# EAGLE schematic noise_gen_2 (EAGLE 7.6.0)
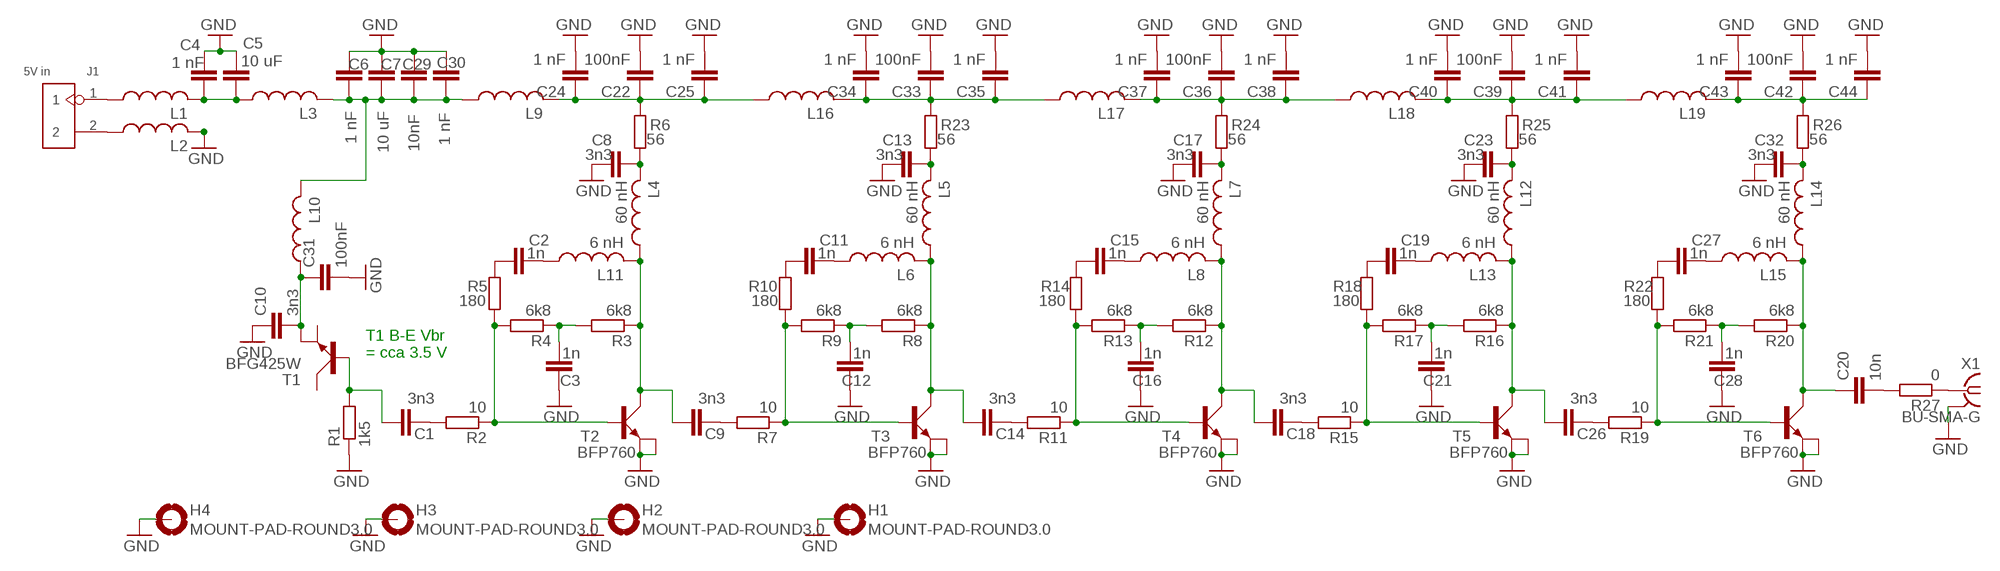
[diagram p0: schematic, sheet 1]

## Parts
C1  3n3  C-EUC0603  [C0603]
C2  1n  C-EUC0603  [C0603]
C3  1n  C-EUC0603  [C0603]
C4  1 nF  C-EUC0603  [C0603]
C5  10 uF  C-EUC1210  [C1210]
C6  1 nF  C-EUC0603  [C0603]
C7  10 uF  C-EUC1210  [C1210]
C8  3n3  C-EUC0603  [C0603]
C9  3n3  C-EUC0603  [C0603]
C10  3n3  C-EUC0603  [C0603]
C11  1n  C-EUC0603  [C0603]
C12  1n  C-EUC0603  [C0603]
C13  3n3  C-EUC0603  [C0603]
C14  3n3  C-EUC0603  [C0603]
C15  1n  C-EUC0603  [C0603]
C16  1n  C-EUC0603  [C0603]
C17  3n3  C-EUC0603  [C0603]
C18  3n3  C-EUC0603  [C0603]
C19  1n  C-EUC0603  [C0603]
C20  10n  C-EUC0603  [C0603]
C21  1n  C-EUC0603  [C0603]
C22  100nF  C-EUC0603  [C0603]
C23  3n3  C-EUC0603  [C0603]
C24  1 nF  C-EUC0603  [C0603]
C25  1 nF  C-EUC0603  [C0603]
C26  3n3  C-EUC0603  [C0603]
C27  1n  C-EUC0603  [C0603]
C28  1n  C-EUC0603  [C0603]
C29  10nF  C-EUC0603  [C0603]
C30  1 nF  C-EUC0603  [C0603]
C31  100nF  C-EUC0603  [C0603]
C32  3n3  C-EUC0603  [C0603]
C33  100nF  C-EUC0603  [C0603]
C34  1 nF  C-EUC0603  [C0603]
C35  1 nF  C-EUC0603  [C0603]
C36  100nF  C-EUC0603  [C0603]
C37  1 nF  C-EUC0603  [C0603]
C38  1 nF  C-EUC0603  [C0603]
C39  100nF  C-EUC0603  [C0603]
C40  1 nF  C-EUC0603  [C0603]
C41  1 nF  C-EUC0603  [C0603]
C42  100nF  C-EUC0603  [C0603]
C43  1 nF  C-EUC0603  [C0603]
C44  1 nF  C-EUC0603  [C0603]
H1  MOUNT-PAD-ROUND3.0  [3,0-PAD]
H2  MOUNT-PAD-ROUND3.0  [3,0-PAD]
H3  MOUNT-PAD-ROUND3.0  [3,0-PAD]
H4  MOUNT-PAD-ROUND3.0  [3,0-PAD]
J1  5V in  DIP-BLACK-MALE-HEADER-VERT(2P-2.54)BIIG_PACKAGE  [H2-2.54_BIIG]
L1  L-US0207/10  [0207/10]
L2  L-US0207/10  [0207/10]
L3  L-USL1812  [L1812]
L4  60 nH  L-USL4516C  [L4516C]
L5  60 nH  L-USL4516C  [L4516C]
L6  6 nH  L-USL3216C  [L3216C]
L7  60 nH  L-USL4516C  [L4516C]
L8  6 nH  L-USL3216C  [L3216C]
L9  L-USL1812  [L1812]
L10  L-USL1812  [L1812]
L11  6 nH  L-USL3216C  [L3216C]
L12  60 nH  L-USL4516C  [L4516C]
L13  6 nH  L-USL3216C  [L3216C]
L14  60 nH  L-USL4516C  [L4516C]
L15  6 nH  L-USL3216C  [L3216C]
L16  L-USL1812  [L1812]
L17  L-USL1812  [L1812]
L18  L-USL1812  [L1812]
L19  L-USL1812  [L1812]
R1  1k5  R-EU_M1206  [M1206]
R2  10  R-EU_R0603  [R0603]
R3  6k8  R-EU_R0603  [R0603]
R4  6k8  R-EU_R0603  [R0603]
R5  180  R-EU_R0603  [R0603]
R6  56  R-EU_R0603  [R0603]
R7  10  R-EU_R0603  [R0603]
R8  6k8  R-EU_R0603  [R0603]
R9  6k8  R-EU_R0603  [R0603]
R10  180  R-EU_R0603  [R0603]
R11  10  R-EU_R0603  [R0603]
R12  6k8  R-EU_R0603  [R0603]
R13  6k8  R-EU_R0603  [R0603]
R14  180  R-EU_R0603  [R0603]
R15  10  R-EU_R0603  [R0603]
R16  6k8  R-EU_R0603  [R0603]
R17  6k8  R-EU_R0603  [R0603]
R18  180  R-EU_R0603  [R0603]
R19  10  R-EU_R0603  [R0603]
R20  6k8  R-EU_R0603  [R0603]
R21  6k8  R-EU_R0603  [R0603]
R22  180  R-EU_R0603  [R0603]
R23  56  R-EU_R0603  [R0603]
R24  56  R-EU_R0603  [R0603]
R25  56  R-EU_R0603  [R0603]
R26  56  R-EU_R0603  [R0603]
R27  0  R-EU_R0603  [R0603]
T1  BFG425W  [SOT343R]
T2  BFP760  [SOT343R]
T3  BFP760  [SOT343R]
T4  BFP760  [SOT343R]
T5  BFP760  [SOT343R]
T6  BFP760  [SOT343R]
X1  BU-SMA-G  [BU-SMA-G]

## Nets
GND: C3.1 C4.1 C5.2 C6.1 C7.2 C8.1 C10.1 C12.1 C13.1 C16.1 C17.1 C21.1 C22.2 C23.1 C24.2 C25.2 C28.1 C29.2 C30.2 C31.2 C32.1 C33.2 C34.2 C35.2 C36.2 C37.2 C38.2 C39.2 C40.2 C41.2 C42.2 C43.2 C44.2 H1.B3,0(MOUNT) H2.B3,0(MOUNT) H3.B3,0(MOUNT) H4.B3,0(MOUNT) L2.2 R1.1 T2.1(E) T2.3(E2) T3.1(E) T3.3(E2) T4.1(E) T4.3(E2) T5.1(E) T5.3(E2) T6.1(E) T6.3(E2) X1.2 X1.3 X1.4 X1.5
N$1: C6.2 C7.1 C29.1 C30.1 L3.2 L9.1 L10.2
N$2: C1.2 R2.2
N$3: R2.1 R4.2 R5.2 T2.2(B)
N$4: C9.2 R7.2
N$5: R7.1 R9.2 R10.2 T3.2(B)
N$6: C13.2 L5.2 R23.1
N$7: J1.1 L1.1
N$8: C4.2 C5.1 L1.2 L3.1
N$9: C3.2 R3.2 R4.1
N$10: J1.2 L2.1
N$11: C8.2 L4.2 R6.1
N$12: C1.1 R1.2 T1.2(B)
N$13: C10.2 C31.1 L10.1 T1.3(E2)
N$14: C20.2 R27.2
N$15: C12.2 R8.2 R9.1
N$16: C11.1 R10.1
N$17: C11.2 L6.1
N$18: C2.1 R5.1
N$19: C14.1 L5.1 L6.2 R8.1 T3.4(C)
N$20: C14.2 R11.2
N$21: R11.1 R13.2 R14.2 T4.2(B)
N$22: C17.2 L7.2 R24.1
N$23: R27.1 X1.1
N$24: C16.2 R12.2 R13.1
N$25: C15.1 R14.1
N$26: C2.2 L11.1
N$27: C15.2 L8.1
N$29: C9.1 L4.1 L11.2 R3.1 T2.4(C)
N$30: C18.1 L7.1 L8.2 R12.1 T4.4(C)
N$31: C18.2 R15.2
N$32: C22.1 C24.1 C25.1 L9.2 L16.1 R6.2
N$33: R15.1 R17.2 R18.2 T5.2(B)
N$34: C23.2 L12.2 R25.1
N$36: C21.2 R16.2 R17.1
N$37: C19.1 R18.1
N$38: C19.2 L13.1
N$39: C26.1 L12.1 L13.2 R16.1 T5.4(C)
N$40: C26.2 R19.2
N$41: R19.1 R21.2 R22.2 T6.2(B)
N$42: C32.2 L14.2 R26.1
N$44: C28.2 R20.2 R21.1
N$45: C27.1 R22.1
N$46: C27.2 L15.1
N$47: C20.1 L14.1 L15.2 R20.1 T6.4(C)
N$48: C33.1 C34.1 C35.1 L16.2 L17.1 R23.2
N$49: C36.1 C37.1 C38.1 L17.2 L18.1 R24.2
N$50: C39.1 C40.1 C41.1 L18.2 L19.1 R25.2
N$51: C42.1 C43.1 C44.1 L19.2 R26.2
Unconnected: T1.1(E) T1.4(C)

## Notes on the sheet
- T1 B-E Vbr
  = cca 3.5 V

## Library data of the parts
C1-C44 = rcl:C-EU: CAPACITOR, European symbol
H1-H4 = holes:MOUNT-PAD-ROUND: MOUNTING PAD, round
J1 = Seeed-OPL-Connector:DIP-BLACK-MALE-HEADER-VERT(2P-2.54): 320020016
L1-L19 = rcl:L-US: INDUCTOR, American symbol
R1-R27 = rcl:R-EU_: RESISTOR, European symbol
T1 = mylib:BFG425W: NXP BFG425W RF BJT, Ft = 25 GHz
T2-T6 = mylib:BFP760: NXP BFG425W RF BJT, Ft = 25 GHz
X1 = con-coax:BU-SMA-G: FEMALE SMA CONNECTOR; OC_FARNELL: unknown; OC_NEWARK: unknown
